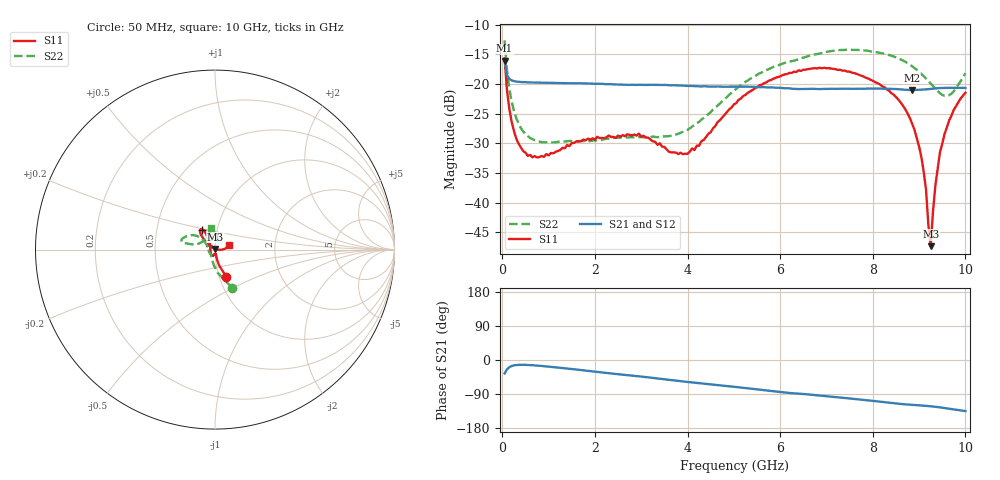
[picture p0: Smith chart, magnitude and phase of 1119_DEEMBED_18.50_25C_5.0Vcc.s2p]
!Hittite Microwave Corp.
!Digital Attenuator/PhaseShifter Rev 1.4.0
!Filename: C:\DATA\DATA\1119_DEEMBED_18.50_25C_5.0Vcc.s2p
!VNA ID: Agilent Technologies,N5224A,MY51441122,A.10.45.03
!Device type:
!2 Port Calibration.
!Temp(C): 25
!Lot Number:
!Serial Number:
!Operator:
!Misc:
!Attenuator:  18.500
# GHZ S DB R 50.0
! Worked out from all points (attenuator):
!   200 points, 50 MHz to 10 GHz, reference 50 ohm
!   highest |S21| = -16.07 dB at 50 MHz (marker M1); lowest = -21.0 dB at 8.85 GHz (marker M2)
!   lowest |S11| = -47.4 dB at 9.25 GHz (marker M3), VSWR 1.01, Z = 50.2 + j0.384 ohm
!   |S11| at or under -10 dB: start of sweep to end of sweep
!   |S22| runs from -29.9 to -12.7 dB; largest |S21 - S12| = 0.00033
!   S11 on the Smith chart (normalised r, x): 50 MHz: 1.08, -0.34; 6.6 GHz: 0.84, +0.19; 10 GHz: 1.17, +0.07
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0.05  -15.67 -67.5  -16.07 -35.5  -16.08 -35.5  -12.67 -65.8
0.1  -20.98 -75.5  -18.46 -24.9  -18.46 -24.9  -17.61 -83.0
0.2  -26.32 -78.7  -19.39 -15.9  -19.39 -15.9  -22.90 -99.7
0.35  -30.05 -78.6  -19.64 -12.9  -19.65 -12.9  -26.68 -113.6
0.55  -32.13 -81.1  -19.74 -13.1  -19.73 -13.1  -28.78 -125.1
1.75  -29.39 -110.3  -19.91 -27.2  -19.91 -27.2  -29.63 -138.7
2.95  -28.38 -124.8  -20.14 -43.0  -20.15 -43.1  -28.97 -157.6
3.4  -30.01 -144.2  -20.17 -49.3  -20.18 -49.4  -28.92 -171.0
4  -31.80 168.4  -20.33 -57.8  -20.34 -57.9  -27.75 164.7
5.05  -23.24 121.7  -20.46 -71.2  -20.48 -71.3  -20.85 140.2
6.6  -17.50 123.2  -20.85 -90.8  -20.86 -90.8  -15.33 153.8
6.7  -17.41 124.0  -20.83 -92.0  -20.85 -92.0  -15.12 154.8
7.5  -17.93 131.1  -20.81 -101.5  -20.82 -101.5  -14.25 164.0
8.35  -21.12 136.6  -20.83 -112.6  -20.83 -112.6  -15.13 167.8
8.85  -26.73 140.2  -21.03 -118.3  -21.03 -118.3  -17.02 167.4
9.1  -34.84 139.0  -20.96 -120.5  -20.97 -120.5  -18.71 165.6
9.15  -37.84 137.2  -20.92 -120.9  -20.94 -121.0  -19.10 164.7
9.25  -47.36 63.2  -20.85 -122.1  -20.87 -122.1  -19.93 161.6
9.35  -37.24 0.9  -20.77 -123.5  -20.79 -123.5  -20.76 156.5
9.45  -31.56 -3.8  -20.69 -125.1  -20.71 -125.0  -21.56 149.0
9.65  -26.13 3.0  -20.66 -128.5  -20.67 -128.5  -21.90 127.0
10  -21.49 19.2  -20.69 -134.8  -20.69 -134.8  -18.20 99.7
